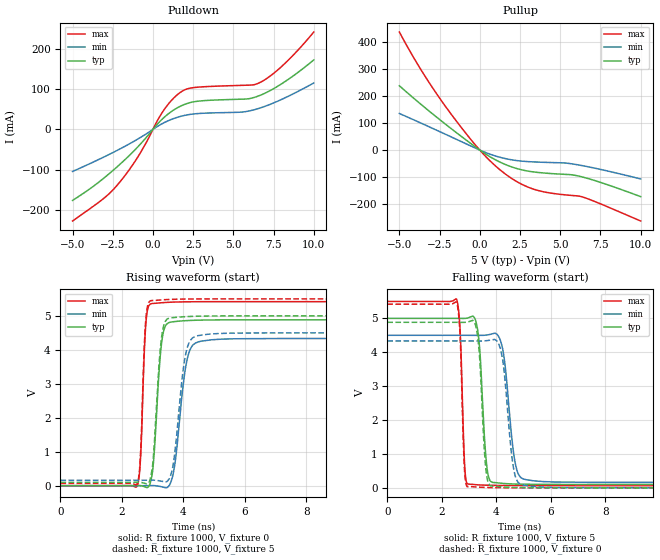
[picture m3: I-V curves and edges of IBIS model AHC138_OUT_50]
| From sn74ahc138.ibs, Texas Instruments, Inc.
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[Model]   AHC138_OUT_50
Model_type  Output
Vref =   0
Rref =   1000
Cref =   15p
Vmeas =   2.5
| variable   typ   min   max
C_comp   3.01pF   2.29pF   4.35pF
| C_pullup   3.29pF   2.43pF   4.35pF
| C_pulldown   2.73pF   2.29pF   3.35pF
[Temperature Range]   40   100   -40
| Ambient temperature   25   85   -40
[Voltage range]   5   4.5   5.5
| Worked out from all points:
|   slope of the pulldown table from 0 to 0.75 V, typ, clamps not added: 23.6 ohm
|   slope of the pullup table from 0 to 0.75 V, typ, clamps not added: 26.1 ohm
|   rising waveform, R_fixture 1000, V_fixture 0: 20-80 % time 205ps typ, 313ps min, 128ps max; typ from 0 V to 4.88 V
|   falling waveform, R_fixture 1000, V_fixture 5: 20-80 % time 202ps typ, 317ps min, 125ps max; typ from 5 V to 0.1 V
|   rising waveform, R_fixture 1000, V_fixture 5: 20-80 % time 207ps typ, 300ps min, 128ps max; typ from 0.1 V to 5 V
|   falling waveform, R_fixture 1000, V_fixture 0: 20-80 % time 192ps typ, 297ps min, 122ps max; typ from 4.88 V to 0 V
[Pulldown]
| AHC138_OUT_50
|   Voltage   I(typ)   I(min)   I(max)
-5V       -176.4mA   -104.5mA   -227.4mA
-3.045V   -120.7mA   -68.43mA   -170.8mA
-2.115V   -88.88mA   -49.82mA   -133.4mA
-875mV    -40.56mA   -22.35mA   -64.35mA
635mV     27.66mA    15.45mA    45.39mA
1.105V    43.12mA    24.17mA    69.94mA
1.6V      55.38mA    31.07mA    88.81mA
2.505V    68.31mA    38.28mA    103.7mA
5.53V     75.05mA    43.01mA    109.4mA
6.59V     83.43mA    52.24mA    115.2mA
8.085V    115.3mA    75.99mA    159.2mA
10V       172.5mA    115.2mA    241.7mA
[Pullup]
| AHC138_OUT_50
|   Voltage   I(typ)   I(min)   I(max)
-5V       238.4mA    135.6mA    437.6mA
-3.51V    162.2mA    96.02mA    283.7mA
-1.84V    82.29mA    50.48mA    137.9mA
10mV      -425.6uA   -267uA     -671.3uA
725mV     -27.91mA   -17.07mA   -45mA
1.435V    -49.54mA   -29.43mA   -81.78mA
2.33V     -68.97mA   -39.22mA   -117.9mA
3.23V     -80.14mA   -43.54mA   -142.6mA
4.31V     -86.53mA   -46.02mA   -158.5mA
5.685V    -91.51mA   -50.76mA   -168.1mA
6.375V    -99.73mA   -57.75mA   -173.7mA
10V       -172.6mA   -106.9mA   -263mA
[Ramp]
| AHC138_OUT_50
| variable   typ   min   max
dV/dt_r   2.96/2.19E-10   2.64/3.23E-10   3.28/1.31E-10
dV/dt_f   2.98/2.12E-10   2.64/3.27E-10   3.31/1.29E-10
R_load = 1000
[Rising Waveform]
| AHC138_OUT_50
R_fixture =   1000
C_fixture =   0
L_fixture =   0
V_fixture =   0
V_fixture_min = 0
V_fixture_max = 0
|   Time   V(typ)   V(min)   V(max)
0s        234.8pV    458.7pV    104.5pV
2.5ns     2.763mV    -142.4uV   -5.453mV
2.61ns    1.109mV    -392.2uV   861.5mV
2.78ns    -43.47mV   651.1uV    4.758V
2.99ns    365.4mV    3.889mV    5.364V
3.315ns   4.342V     -36.73mV   5.387V
3.725ns   4.833V     638.4mV    5.406V
4.175ns   4.863V     3.893V     5.414V
4.92ns    4.879V     4.295V     5.418V
50ns      4.884V     4.333V     5.419V
[Falling Waveform]
| AHC138_OUT_50
R_fixture =   1000
C_fixture =   0
L_fixture =   0
V_fixture =   5
V_fixture_min = 4.5
V_fixture_max = 5.5
|   Time   V(typ)   V(min)   V(max)
0s        5V         4.5V       5.5V
2.55ns    5V         4.5V       5.554V
2.965ns   5.013V     4.5V       110.1mV
3.315ns   4.679V     4.498V     89.73mV
3.645ns   707.9mV    4.508V     78.03mV
3.875ns   159.4mV    4.548V     73.59mV
4.25ns    131.2mV    4.048V     69.66mV
4.755ns   111.4mV    537.6mV    67.38mV
5.37ns    103.6mV    207.9mV    66.35mV
50ns      99.57mV    160.9mV    65.74mV
[Rising Waveform]
| AHC138_OUT_50
R_fixture =   1000
C_fixture =   0
L_fixture =   0
V_fixture =   5
V_fixture_min = 4.5
V_fixture_max = 5.5
|   Time   V(typ)   V(min)   V(max)
0s        99.57mV    160.9mV    65.74mV
2.5ns     102.2mV    160.8mV    64.87mV
2.605ns   100.9mV    160.6mV    907.1mV
2.77ns    62.21mV    161.5mV    4.785V
2.94ns    264.2mV    164mV      5.446V
3.285ns   4.315V     133.2mV    5.469V
3.585ns   4.94V      297.6mV    5.484V
4.11ns    4.978V     4.003V     5.495V
4.785ns   4.995V     4.457V     5.499V
50ns      5V         4.5V       5.5V
[Falling Waveform]
| AHC138_OUT_50
R_fixture =   1000
C_fixture =   0
L_fixture =   0
V_fixture =   0
V_fixture_min = 0
V_fixture_max = 0
|   Time   V(typ)   V(min)   V(max)
0s        4.884V     4.333V     5.419V
2.545ns   4.884V     4.333V     5.473V
2.935ns   4.891V     4.333V     34.49mV
3.31ns    4.529V     4.332V     22.62mV
3.605ns   680.2mV    4.338V     12.48mV
3.805ns   53.3mV     4.361V     8.47mV
4.23ns    28.2mV     3.818V     3.886mV
4.695ns   11.55mV    361mV      1.761mV
5.285ns   4.154mV    47.6mV     687uV
50ns      -6.597nV   -1.418nV   -2.979nV
